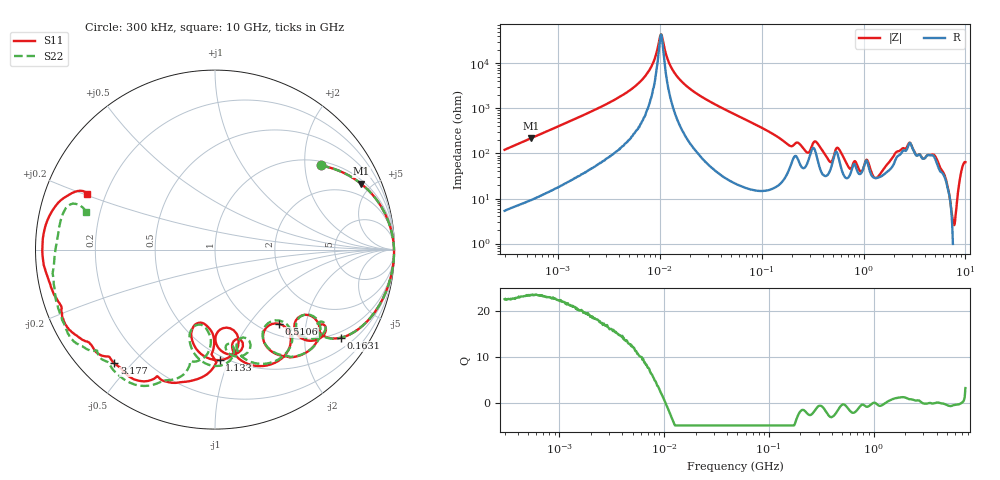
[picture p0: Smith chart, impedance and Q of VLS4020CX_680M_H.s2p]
! S-Parameter Data Generated by TDK Corporation
! Copyright(C) 2024 TDK Corporation.
! All Rights Reserved.
! TDK P/N: VLS4020CX-680M-H (SMD / SMT Inductor (Coil))
! Property: L=68uH at 1MHz
! Size(LxWxT): 4x4x2mm
! Model Type: s2p (Touchstone File Format Version 1.0)
! Frequency: DC=Yes Start=0.3MHz Stop=10000MHz 802points Log-sweep
! Model Generated on May 28, 2024
! Terms and conditions regarding TDK Simulation Models:
! 1)This simulation model is being provided solely for informational
!  purposes. Please refer to the specifications of the products in
!  terms of detailed characteristics of such products.
! 2)In no event shall TDK Corporation of any of its subsidiaries be
!  liable for any loss or damage arising, directly or indirectly,
!  from any information contained in this simulation model, including,
!  but not limited to loss or damages arising from any inaccuracies,
!  omissions or errors in connection with such information.
! 3)Any and all copyrights on this simulation model are owned by
!  TDK Corporation.  Duplication or redistribution of this simulation
!  model without prior written permission from TDK Corporation
!  is prohibited.
! 4)This simulation model is subject to any modification or change
!  without any prior notice.
! 5)Neither TDK Corporation nor any of its subsidiaries shall make any
!  warranty, express or implied, including but not limited to the
!  correctness, implied warranties of merchantability and fitness for
!  a particular purpose with respect to this simulation models.
! 6)The use of this simulation model shall be deemed to have consented
!  to the terms and conditions hereof.
! Port Assignments:
!  1 ---@@@--- 2
! Applicable Conditions:
!  Temperature = 25 degC
!  DC Bias Current = 0 A
!  Small Signal Operation
# Hz S MA R 50
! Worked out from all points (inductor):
!   801 points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, 300 kHz to 10 GHz, reference 50 ohm
!   read as one part in series: L = 63.8 uH near 318.3 kHz
!   highest Q = 23.6 at 542.3 kHz (marker M1), where L = 63.5 uH
!   self-resonance near 10.27 MHz
!   S11 on the Smith chart (normalised r, x): 300 kHz: 1.11, +2.42; 163.1 MHz: 0.81, -2.96; 510.6 MHz: 1.20, -1.42; 1.133 GHz: 0.47, -0.93; 3.177 GHz: 0.10, -0.45; 10 GHz: 0.13, +0.20
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300000  0.7538 38.4  0.6244 -49.0  0.6245 -49.0  0.754 38.4
542347  0.8935 24.2  0.4125 -63.3  0.4126 -63.3  0.8936 24.2
1713600  0.9823 8.1  0.144 -79.0  0.1439 -78.9  0.9823 8.1
6127430  0.9968 1.2  0.02812 -83.1  0.02811 -82.9  0.9968 1.2
8246826  0.9974 0.1  0.0119 -78.0  0.01186 -77.9  0.9975 0.1
9671944  0.9977 -0.4  0.003994 -55.1  0.003989 -55.3  0.9977 -0.4
1.03845e7  0.9977 -0.7  0.002282 10.6  0.002289 10.4  0.9978 -0.7
1.289893e7  0.9977 -1.5  0.01202 78.0  0.01203 78.1  0.9978 -1.5
1.763281e7  0.9973 -2.8  0.02947 82.9  0.02948 82.9  0.9974 -2.8
5.477226e7  0.9871 -11.2  0.1338 77.2  0.1338 77.1  0.9871 -11.2
1.630679e8  0.855 -35.1  0.4239 47.5  0.424 47.5  0.8516 -35.3
3.126428e8  0.6553 -34.5  0.3987 4.9  0.3988 4.9  0.6598 -34.1
3.970454e8  0.7307 -55.3  0.5195 20.2  0.5196 20.2  0.7301 -54.9
5.105874e8  0.5468 -49.1  0.5046 -12.8  0.5047 -12.8  0.533 -47.8
6.15965e8  0.7014 -67.6  0.5118 4.4  0.5119 4.4  0.6984 -65.2
1.133369e9  0.6165 -87.6  0.5059 -30.6  0.5062 -30.7  0.6442 -92.6
1.767019e9  0.4416 -94.0  0.532 -88.6  0.5323 -88.7  0.4649 -94.4
2.264206e9  0.7534 -102.3  0.2733 -112.2  0.2737 -112.2  0.6529 -102.4
3.177248e9  0.8459 -131.6  0.1439 -96.7  0.1439 -96.9  0.8783 -130.1
5.526371e9  0.923 -157.4  0.08149 -98.3  0.08109 -98.4  0.9411 -151.7
7.428478e9  0.9615 -178.1  0.07463 -118.2  0.07442 -118.1  0.9006 -174.9
1e10  0.7752 156.5  0.05694 -124.7  0.05704 -124.7  0.7474 163.6
